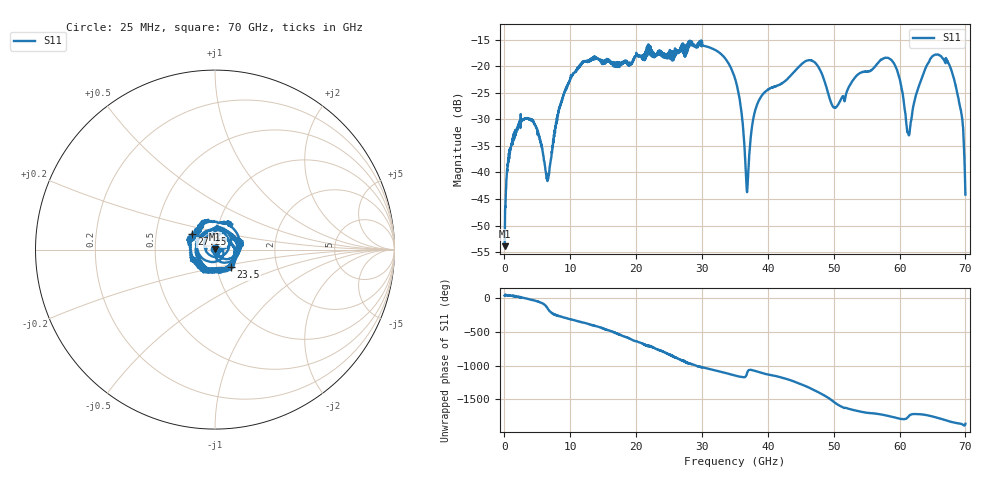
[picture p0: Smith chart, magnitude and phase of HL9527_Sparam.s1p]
! 1/10/2024 10:50:31 AM
! H:\PROTOTYPE_DATA\110GHZ-ATTN\TERM\3094.S1P
! CHANNEL.1
! TR.MEASUREMENT
! CORRECTED.DATA
! RF.CORRECTION: FULL.TWO.PORT.CAL.PORT.1.2
! AVERAGING: 1 PointByPoint
! IF.BANDWIDTH: 1KHZ
! SWEEPTYPE:  FREQ.SWEEP(Linear)
! Reference Plane Port Info
! PORT:  PORT1
! DISTANCE:  0  m
! TIME:  0  s
! PHASE.OFFSET:  0 °
! LOSS:  0  dB
! REF.LOSS:  0  dB
! REF.FREQ:  0  Hz
! Power Info
! POWER:  -10  dBm
! EFF.POWER:  -10  dBm
! POWER(>54G):  -10  dBm
! EFF.POWER(>54G):  -10  dBm
! SOURCE.ATTEN:  0  dB
! TEST.ATTEN:  0  dB
# GHZ S RI R 50.0
! FREQ.GHZ  S11RE  S11IM
!; PortSelection: Port_1
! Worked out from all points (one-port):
!   2800 points, 25 MHz to 70 GHz, reference 50 ohm
!   lowest |S11| = -53.9 dB at 25 MHz (marker M1), VSWR 1.00, Z = 50.1 + j0.141 ohm
!   |S11| at or under -10 dB: start of sweep to end of sweep
!   S11 on the Smith chart (normalised r, x): 25 MHz: 1.00, +0.00; 23.5 GHz: 1.17, -0.23; 27.25 GHz: 0.76, +0.13; 70 GHz: 1.01, -0.01
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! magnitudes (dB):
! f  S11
! 25 MHz  -53.9
! 650 MHz  -37.0
! 1.95 GHz  -31.7
! 4.45 GHz  -30.4
! 6.55 GHz  -41.3
! 8.775 GHz  -26.3
! 12.05 GHz  -19.0
! 17.52 GHz  -19.9
! 23.5 GHz  -17.6
! 26.27 GHz  -17.5
! 27.25 GHz  -16.2
! 32.17 GHz  -17.0
! 35.02 GHz  -22.3
! 35.9 GHz  -27.7
! 36.85 GHz  -43.7
! 38.58 GHz  -26.6
! 43.77 GHz  -21.4
! 47.02 GHz  -19.2
! 50.15 GHz  -27.8
! 52.52 GHz  -23.4
! 58.6 GHz  -18.7
! 59.95 GHz  -22.1
! 61.27 GHz  -32.5
! 63.92 GHz  -20.4
! 66.17 GHz  -18.0
! 68.75 GHz  -25.0
! 69.45 GHz  -29.4
! 70 GHz  -44.2
